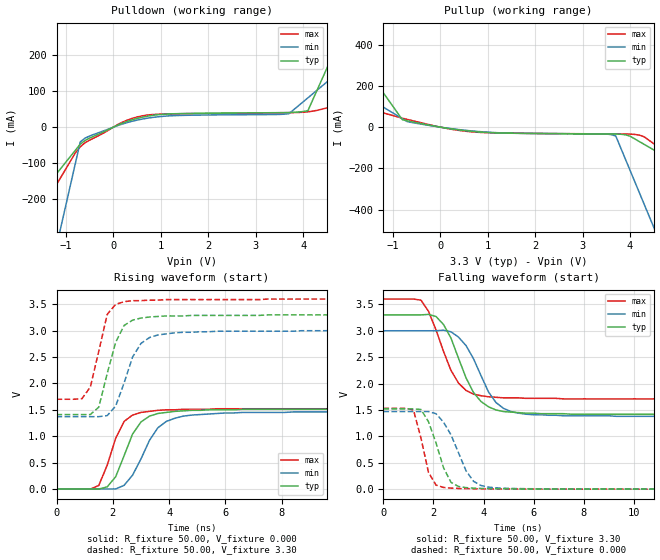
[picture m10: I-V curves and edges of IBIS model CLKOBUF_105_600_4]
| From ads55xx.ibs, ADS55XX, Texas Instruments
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|   Model CLKOBUF_105_600_4
[Model]   CLKOBUF_105_600_4
Model_type   Output
Polarity   Non-Inverting
Vmeas =   1.65V
C_comp   2pf   2pf   2pf
[Temperature Range]   50.00   0.10k   -20.00
[Voltage Range]   3.30V   3.00V   3.60V
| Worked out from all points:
|   slope of the pulldown table from 0 to 0.495 V, typ, clamps not added: 20.4 ohm
|   slope of the pullup table from 0 to 0.495 V, typ, clamps not added: 30.4 ohm
|   rising waveform, R_fixture 50.00, V_fixture 0.000: 20-80 % time 765ps typ, 889ps min, 654ps max; typ from 0 V to 1.51 V
|   rising waveform, R_fixture 50.00, V_fixture 3.30: 20-80 % time 622ps typ, 715ps min, 495ps max; typ from 1.41 V to 3.3 V
|   falling waveform, R_fixture 50.00, V_fixture 3.30: 20-80 % time 1.05ns typ, 1.05ns min, 976ps max; typ from 3.3 V to 1.41 V
|   falling waveform, R_fixture 50.00, V_fixture 0.000: 20-80 % time 665ps typ, 865ps min, 460ps max; typ from 1.52 V to 0.001 V
[Pulldown]
| voltage   I(typ)   I(min)   I(max)
-3.3V     -476.5mA   -1.554A    -628.5mA
-2.1V     -278.5mA   -855.7mA   -360.9mA
-1.7V     -212.5mA   -623mA     -271.7mA
-1.5V     -179.5mA   -506.6mA   -227.1mA
-1V       -97.01mA   -215.8mA   -115.6mA
-700mV    -47.51mA   -41.29mA   -54.99mA
400mV     20.76mA    16.58mA    24.57mA
3.7V      40.69mA    37.5mA     40.52mA
4.1V      45.88mA    81.74mA    42.8mA
4.9V      282.8mA    170.2mA    66.97mA
5.9V      578.9mA    280.8mA    100.2mA
6.6V      786.1mA    358.2mA    123.5mA
[Pullup]
| voltage   I(typ)   I(min)   I(max)
-3.3V     847.2mA    389.8mA    202.8mA
-2.3V     522.7mA    250.2mA    139mA
-2.1V     457.8mA    222.3mA    126.2mA
-800mV    35.97mA    40.8mA     43.27mA
-600mV    25.94mA    22.4mA     32.05mA
700mV     -21.1mA    -19.17mA   -23.42mA
3.6V      -33.08mA   -35.96mA   -32.73mA
3.7V      -33.33mA   -43.17mA   -32.85mA
4V        -43.63mA   -208.9mA   -33.79mA
4.2V      -70.29mA   -319.4mA   -38.78mA
4.5V      -110.3mA   -485.1mA   -80.14mA
6.6V      -390.2mA   -1.645A    -428.7mA
[Ramp]
| variable   typ   min   max
dV/dt_r   0.91/0.72n   0.88/0.88n   0.91/0.61n
dV/dt_f   1.13/1.02n   0.97/1.03n   1.14/0.94n
R_load = 50.00
[Rising Waveform]
R_fixture = 50.00
V_fixture = 0.000
V_fixture_min = 0.000
V_fixture_max = 0.000
| time   V(typ)   V(min)   V(max)
0s        25.41nV    34.58nV    50.27nV
1.5ns     -3.54mV    29.9uV     65.18mV
1.8ns     39.32mV    -2.05mV    450mV
2.1ns     230mV      -1.07mV    960mV
2.4ns     630mV      68.1mV     1.28V
2.7ns     1.04V      260mV      1.4V
3ns       1.27V      570mV      1.45V
3.6ns     1.43V      1.16V      1.49V
4.5ns     1.48V      1.38V      1.51V
15ns      1.51V      1.46V      1.52V
[Rising Waveform]
R_fixture = 50.00
V_fixture = 3.30
V_fixture_min = 3.00
V_fixture_max = 3.60
| time   V(typ)   V(min)   V(max)
0s        1.41V      1.37V      1.7V
900ps     1.41V      1.37V      1.71V
1.2ns     1.41V      1.37V      1.93V
1.5ns     1.55V      1.37V      2.61V
1.8ns     2.19V      1.39V      3.31V
2.1ns     2.78V      1.57V      3.5V
2.4ns     3.1V       2.01V      3.55V
3ns       3.24V      2.76V      3.57V
3.6ns     3.27V      2.92V      3.58V
15ns      3.3V       3V         3.6V
[Falling Waveform]
R_fixture = 50.00
V_fixture = 3.30
V_fixture_min = 3.00
V_fixture_max = 3.60
| time   V(typ)   V(min)   V(max)
0s        3.3V       3V         3.6V
1.5ns     3.3V       3V         3.58V
2.1ns     3.27V      3V         3.02V
2.7ns     2.86V      2.98V      2.25V
3ns       2.48V      2.88V      2.01V
3.6ns     1.83V      2.47V      1.8V
4.2ns     1.56V      1.84V      1.75V
4.5ns     1.5V       1.64V      1.74V
5.4ns     1.45V      1.44V      1.73V
15ns      1.41V      1.38V      1.71V
[Falling Waveform]
R_fixture = 50.00
V_fixture = 0.000
V_fixture_min = 0.000
V_fixture_max = 0.000
| time   V(typ)   V(min)   V(max)
0s        1.52V      1.47V      1.53V
1.2ns     1.52V      1.47V      1.5V
1.5ns     1.51V      1.47V      970mV
1.8ns     1.28V      1.47V      320mV
2.1ns     880mV      1.43V      78.51mV
2.4ns     410mV      1.27V      33.07mV
2.7ns     130mV      1.03V      20.61mV
3.3ns     30.48mV    350mV      10.62mV
4.2ns     11.53mV    39.77mV    6.19mV
15ns      1mV        1.34mV     1.02mV
